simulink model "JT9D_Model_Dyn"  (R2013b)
settings: Solver=ode4  StartTime=0.0  StopTime=30  FixedStep=0.04  RelTol=1e-3
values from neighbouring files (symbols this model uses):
  MWS = setup_Inputs(MWS)    [JT9D_setup_everything_Dyn.m]    (also in JT9D_setup_everything_SS.m; Tsetup_Ambient.m = MWS; GasTurbine_Dyn_setup_everything.m = setup_Duct(MWS))
libraries: Lib_Turbo_Duct_TMATS x5, Lib_Turbo_Compressor_TMATS x3, Lib_Solve_OuterLoopIntegrator_TMATS x2, Lib_Turbo_Shaft_TMATS x2, Lib_Turbo_TurbineNPSS_TMATS x2, Lib_Turbo_Nozzle_TMATS x2, Lib_Cntrl_SimplePIcontroller_TMATS x1, Lib_Solve_IterNRSolverJC_TMATS x1, Lib_Turbo_Burner_TMATS x1, Lib_Turbo_Inlet_TMATS x1, Lib_Turbo_Splitter_TMATS x1

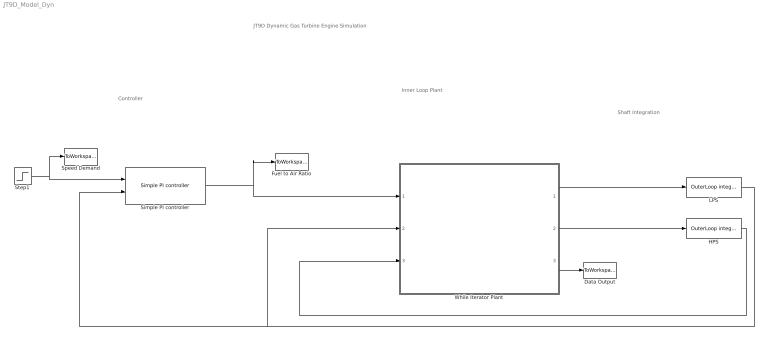
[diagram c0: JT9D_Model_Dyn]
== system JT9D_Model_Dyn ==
  note: JT9D Dynamic Gas Turbine Engine Simulation
  note: Controller
  note: Inner Loop Plant
  note: Shaft Integration
  Data Output : ToWorkspace  VariableName=Plant_Data  SampleTime=-1  SaveFormat=Timeseries
  Fuel to Air Ratio : ToWorkspace  VariableName=FAR  SampleTime=-1  SaveFormat=Timeseries
  HPS : Lib_Solve_OuterLoopIntegrator_TMATS/OuterLoop integrator  OL_IC_M=MWS.Input.HP_Shaft
  LPS : Lib_Solve_OuterLoopIntegrator_TMATS/OuterLoop integrator  OL_IC_M=MWS.Input.LP_Shaft
  Simple PI controller : Lib_Cntrl_SimplePIcontroller_TMATS/Simple PI controller  Kp_M=0.000008  Ki_M=0.00001  PI_IC_M=MWS.Input.FARin
  Speed Demand : ToWorkspace  VariableName=Nf_dmd  SampleTime=-1  SaveFormat=Timeseries
  Step1 : Step  Time=15  Before=MWS.Input.LP_Shaft  After=MWS.Input.LP_Shaft -200  SampleTime=0
  While Iterator Plant : Subsystem  TreatAsAtomicUnit=on
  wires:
  While Iterator Plant/1(LPS_Ndot) -> LPS/1
  While Iterator Plant/2(HPS_Ndot) -> HPS/1
  LPS/1 -> Simple PI controller/2, While Iterator Plant/2(LPS_NmechIn)
  HPS/1 -> While Iterator Plant/3(HPS_NmechIn)
  Simple PI controller/1 -> Fuel to Air Ratio/1, While Iterator Plant/1(FAR_Wf)
  Step1/1 -> Speed Demand/1, Simple PI controller/1
  While Iterator Plant/3(Plant_Data) -> Data Output/1

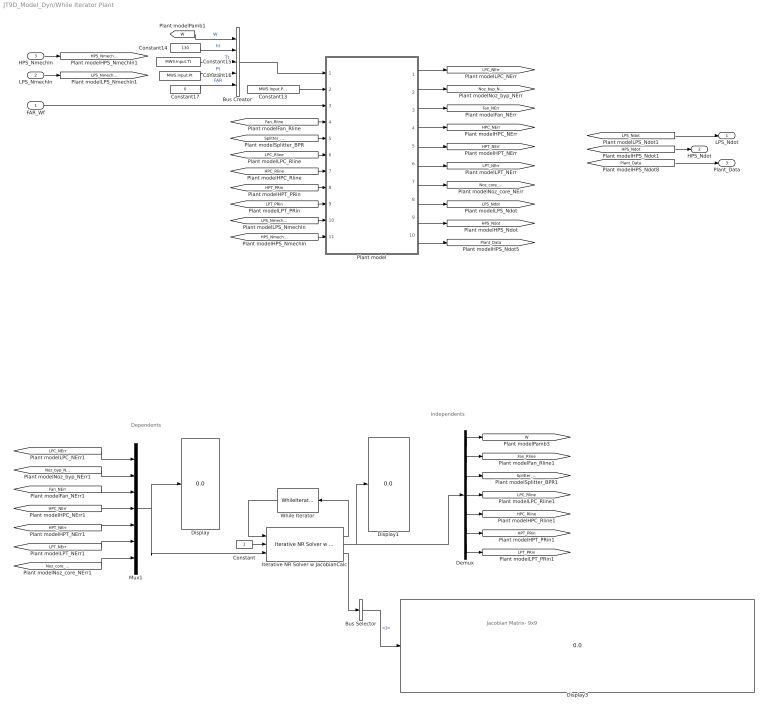
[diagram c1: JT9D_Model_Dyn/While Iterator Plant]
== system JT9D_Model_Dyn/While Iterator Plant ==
  note: Jacobian Matrix- 9x9
  note: Dependents
  note: Independents
  FAR_Wf : Inport
  LPS_NmechIn : Inport  Port=2
  HPS_NmechIn : Inport  Port=3
  Bus Creator : BusCreator  Inputs=5
  Bus Selector : BusSelector  OutputSignals=J
  Constant : Constant
  Constant13 : Constant  Value=MWS.Input.Pamb
  Constant14 : Constant  Value=130
  Constant15 : Constant  Value=MWS.Input.Tt
  Constant16 : Constant  Value=MWS.Input.Pt
  Constant17 : Constant  Value=0
  Demux : Demux  Outputs=7
  Display : Display
  Display1 : Display
  Display3 : Display
  Iterative NR Solver w JacobianCalc : Lib_Solve_IterNRSolverJC_TMATS/Iterative NR Solver w JacobianCalc  SJac_Per_M=[0.05 0.05 0.05 0.05 0.05 0.05 0.05]  SNR_IC_M=MWS.Input.NRICDyn  SNR_DX_M=5  SJacobianAttempts_M=20  Cond_Limits_M=0.0001
  Mux1 : Mux  Inputs=7
  Plant model : Subsystem
  While Iterator : WhileIterator  WhileBlockType=do-while  ShowIterationPort=on
  LPS_Ndot : Outport
  HPS_Ndot : Outport  Port=2
  Plant_Data : Outport  Port=3
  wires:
  [W] -> Bus Creator/1  "W"
  Bus Creator/1 -> Plant model/1(Input GPC)
  Constant17/1 -> Bus Creator/5  "FAR"
  Constant15/1 -> Bus Creator/3  "Tt"
  Constant16/1 -> Bus Creator/4  "Pt"
  Constant14/1 -> Bus Creator/2  "ht"
  Constant13/1 -> Plant model/2(Pamb)
  FAR_Wf/1 -> Plant model/3(FAR_dmd)
  [Fan_Rline] -> Plant model/4(Fan_Rline)
  [Splitter_BPR] -> Plant model/5(Splitter_BPR)
  [LPC_Rline] -> Plant model/6(LPC_Rline)
  [HPC_Rline] -> Plant model/7(HPC_Rline)
  [HPT_PRin] -> Plant model/8(HPT_PRin)
  [LPT_PRin] -> Plant model/9(LPT_PRin)
  [LPS_NmechIn] -> Plant model/10(LPS_NmechIn)
  [HPS_NmechIn] -> Plant model/11(HPS_NmechIn)
  Plant model/1(LPC_NErr) -> [LPC_NErr]
  Plant model/2(Noz_byp_NErr) -> [Noz_byp_NErr]
  Plant model/3(Fan_NErr) -> [Fan_NErr]
  Plant model/4(HPC_NErr) -> [HPC_NErr]
  Plant model/5(HPT_NErr) -> [HPT_NErr]
  Plant model/6(LPT_NErr) -> [LPT_NErr]
  Plant model/7(Noz_core_NErr) -> [Noz_core_NErr]
  Plant model/8(LPS_Ndot) -> [LPS_Ndot]
  Plant model/9(HPS_Ndot) -> [HPS_Ndot]
  Demux/1 -> [W]
  Demux/7 -> [LPT_PRin]
  Demux/5 -> [HPC_Rline]
  Demux/6 -> [HPT_PRin]
  Demux/4 -> [LPC_Rline]
  Demux/2 -> [Fan_Rline]
  Demux/3 -> [Splitter_BPR]
  [Fan_NErr] -> Mux1/3
  [HPC_NErr] -> Mux1/4
  [Noz_byp_NErr] -> Mux1/2
  [HPT_NErr] -> Mux1/5
  [LPC_NErr] -> Mux1/1
  [LPT_NErr] -> Mux1/6
  [Noz_core_NErr] -> Mux1/7
  Iterative NR Solver w JacobianCalc/3 -> Bus Selector/1
  Mux1/1 -> Iterative NR Solver w JacobianCalc/3, Display/1
  Bus Selector/1 -> Display3/1  "<J>"
  Iterative NR Solver w JacobianCalc/2 -> Demux/1, Display1/1
  Iterative NR Solver w JacobianCalc/1 -> While Iterator/1
  HPS_NmechIn/1 -> [HPS_NmechIn]
  LPS_NmechIn/1 -> [LPS_NmechIn]
  [LPS_Ndot] -> LPS_Ndot/1
  [HPS_Ndot] -> HPS_Ndot/1
  Plant model/10(Plant_Data) -> [Plant_Data]
  [Plant_Data] -> Plant_Data/1
  Constant/1 -> Iterative NR Solver w JacobianCalc/2
  While Iterator/1 -> Iterative NR Solver w JacobianCalc/1

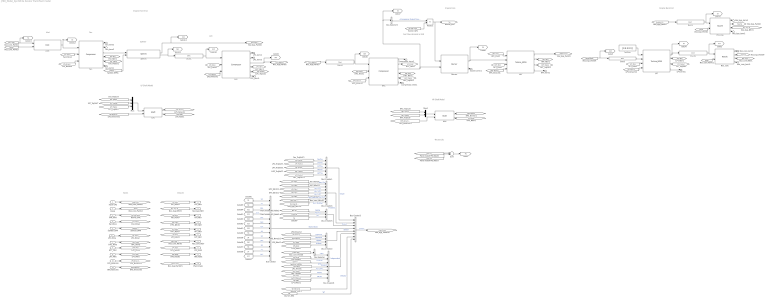
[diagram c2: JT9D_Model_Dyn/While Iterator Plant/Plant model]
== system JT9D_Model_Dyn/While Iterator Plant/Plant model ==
  note: LP Shaft Model
  note: Inputs
  note: Outputs
  note: Engine Core
  note: HP Shaft Model
  note: Engine Back End
  note: Engine Front End
  note: Fuel Flow demand as FAR
  note: Inlet
  note: Fan
  note: Splitter
  note: LPC
  note: Thrust Calc
  Input GPC : Inport
  Pamb : Inport  Port=2
  FAR_dmd : Inport  Port=3
  Fan_Rline : Inport  Port=4
  Splitter_BPR : Inport  Port=5
  LPC_Rline : Inport  Port=6
  HPC_Rline : Inport  Port=7
  HPT_PRin : Inport  Port=8
  LPT_PRin : Inport  Port=9
  LPS_NmechIn : Inport  Port=10
  HPS_NmechIn : Inport  Port=11
  Burner : Lib_Turbo_Burner_TMATS/Burner  LHV_M=18400  dPnormBurner_M=MWS.Burn.dP  Eff_M=0.994
  Burner_term1 : Terminator
  Bus Creator : BusCreator  Inputs=13
  Bus Creator1 : BusCreator  Inputs=5
  Bus Creator2 : BusCreator
  Bus Creator3 : BusCreator  Inputs=8
  Bus Creator4 : BusCreator  Inputs=7
  Bus Creator5 : BusCreator  Inputs=3
  Bus Creator6 : BusCreator  Inputs=7
  Bus Selector : BusSelector  OutputSignals=W
  Bus Selector5 : BusSelector  OutputSignals=Compressor Output Flow; WOut[pps]
  Compressor_term1 : Terminator
  Compressor_term2 : Terminator
  Duct1 : Lib_Turbo_Duct_TMATS/Duct  dP_M=MWS.Duct.dP1
  Duct2 : Lib_Turbo_Duct_TMATS/Duct  dP_M=MWS.Duct.dP2
  Duct3 : Lib_Turbo_Duct_TMATS/Duct  dP_M=MWS.Duct.dP3
  Duct4 : Lib_Turbo_Duct_TMATS/Duct  dP_M=MWS.Duct.dP4
  Duct5 : Lib_Turbo_Duct_TMATS/Duct  dP_M=MWS.Duct.dP5
  Fan : Lib_Turbo_Compressor_TMATS/Compressor  X_C_RlineVec_M=MWS.FAN.RlineVec  Y_C_NcVec_M=MWS.FAN.NcVec  T_C_Map_WcArray_M=MWS.FAN.WcArray  T_C_Map_PRArray_M=MWS.FAN.PRArray  T_C_Map_EffArray_M=MWS.FAN.EffArray  s_C_Nc_M=MWS.FAN.s_Nc  s_C_Wc_M=MWS.FAN.s_Wc  s_C_PR_M=MWS.FAN.s_PR  s_C_Eff_M=MWS.FAN.s_eff  CBLDEN_M=off  C_CBD_M=0  C_CBFht_M=0.5  C_CBFPt_M=0.5  FBLDEN_M=off  C_FBD_M=0  C_BFht_M=0.5  C_BFPt_M=0.5  X_C_WcSurgeVec_M=[0 5000]  T_C_PRSurgeVec_M=[30 30]  iDesign_M=MWS.iDes  NcDes_M=1  EffDes_M=0.8675  PRDes_M=1.645  RlineDes_M=2.3706  FVar_M='iDesScalars.mat'  SVar_M=gcb  NcNm_M='_C_Nc'  WcNm_M='_C_Wc'  PRNm_M='_C_PR'  EffNm_M='_C_Eff'
  Fan_term1 : Terminator
  Fan_term2 : Terminator
  Fan_term3 : Terminator
  HPC : Lib_Turbo_Compressor_TMATS/Compressor  X_C_RlineVec_M=MWS.HPC.RlineVec  Y_C_NcVec_M=MWS.HPC.NcVec  T_C_Map_WcArray_M=MWS.HPC.WcArray  T_C_Map_PRArray_M=MWS.HPC.PRArray  T_C_Map_EffArray_M=MWS.HPC.EffArray  s_C_Nc_M=MWS.HPC.s_Nc  s_C_Wc_M=MWS.HPC.s_Wc  s_C_PR_M=MWS.HPC.s_PR  s_C_Eff_M=MWS.HPC.s_eff  CBLDEN_M=off  C_CBD_M=0  C_CBFht_M=0.5  C_CBFPt_M=0.5  FBLDEN_M=on  C_FBD_M=MWS.HPC.Fbld  C_BFht_M=MWS.HPC.Fblde  C_BFPt_M=MWS.HPC.Fbldp  X_C_WcSurgeVec_M=[0 200]  T_C_PRSurgeVec_M=[30 30]  iDesign_M=MWS.iDes  NcDes_M=0.995  EffDes_M=.8651  PRDes_M=5.609  RlineDes_M=2.0424  FVar_M='iDesScalars.mat'  SVar_M=gcb  NcNm_M='_C_Nc'  WcNm_M='_C_Wc'  PRNm_M='_C_PR'  EffNm_M='_C_Eff'
  HPS : Lib_Turbo_Shaft_TMATS/Shaft  Shaft_Inertia_M=MWS.Shaft.Iner_hp
  HPT : Lib_Turbo_TurbineNPSS_TMATS/Turbine_NPSS  X_T_PRVec_M=MWS.HPT.PRVec  Y_T_NcVec_M=MWS.HPT.NcVec  T_T_Map_WcArray_M=MWS.HPT.WcArray  T_T_Map_EffArray_M=MWS.HPT.EffArray  s_T_Nc_M=MWS.HPT.s_Nc  s_T_Wc_M=MWS.HPT.s_Wc  s_T_PR_M=MWS.HPT.s_PR  s_T_Eff_M=MWS.HPT.s_eff  CFlwEn_M=on  T_CoolFlwPos_M=MWS.HPT.Cool  iDesign_M=MWS.iDes  NcDes_M=99.031  EffDes_M=.9133  PRDes_M=4.930  NDes_M=7390  FVar_M='iDesScalars.mat'  SVar_M=gcb  NcNm_M='_C_Nc'  WcNm_M='_C_Wc'  PRNm_M='_C_PR'  EffNm_M='_C_Eff'
  HPT_term1 : Terminator
  Inlet : Lib_Turbo_Inlet_TMATS/Inlet  eRambase_M=MWS.Inlet.eRamBase  X_eRamVec_M=MWS.Inlet.eRamVec  T_eRamtbl_M=MWS.Inlet.eRamtbl
  LPC : Lib_Turbo_Compressor_TMATS/Compressor  X_C_RlineVec_M=MWS.LPC.RlineVec  Y_C_NcVec_M=MWS.LPC.NcVec  T_C_Map_WcArray_M=MWS.LPC.WcArray  T_C_Map_PRArray_M=MWS.LPC.PRArray  T_C_Map_EffArray_M=MWS.LPC.EffArray  s_C_Nc_M=MWS.LPC.s_Nc  s_C_Wc_M=MWS.LPC.s_Wc  s_C_PR_M=MWS.LPC.s_PR  s_C_Eff_M=MWS.LPC.s_eff  CBLDEN_M=off  C_CBD_M=0  C_CBFht_M=0.5  C_CBFPt_M=0.5  FBLDEN_M=off  C_FBD_M=0  C_BFht_M=0.5  C_BFPt_M=0.5  X_C_WcSurgeVec_M=[0 200]  T_C_PRSurgeVec_M=[30 30]  iDesign_M=MWS.iDes  NcDes_M=0.993  EffDes_M=.8683  PRDes_M=2.488  RlineDes_M=1.7664  FVar_M='iDesScalars.mat'  SVar_M=gcb  NcNm_M='_C_Nc'  WcNm_M='_C_Wc'  PRNm_M='_C_PR'  EffNm_M='_C_Eff'
  LPC_term1 : Terminator
  LPC_term2 : Terminator
  LPC_term3 : Terminator
  LPS : Lib_Turbo_Shaft_TMATS/Shaft  Shaft_Inertia_M=MWS.Shaft.Iner_lp
  LPT : Lib_Turbo_TurbineNPSS_TMATS/Turbine_NPSS  X_T_PRVec_M=MWS.LPT.PRVec  Y_T_NcVec_M=MWS.LPT.NcVec  T_T_Map_WcArray_M=MWS.LPT.WcArray  T_T_Map_EffArray_M=MWS.LPT.EffArray  s_T_Nc_M=MWS.LPT.s_Nc  s_T_Wc_M=MWS.LPT.s_Wc  s_T_PR_M=MWS.LPT.s_PR  s_T_Eff_M=MWS.LPT.s_eff  CFlwEn_M=off  T_CoolFlwPos_M=0  iDesign_M=MWS.iDes  NcDes_M=105.038  EffDes_M=.9323  PRDes_M=6.420  NDes_M=3667.6  FVar_M='iDesScalars.mat'  SVar_M=gcb  NcNm_M='_C_Nc'  WcNm_M='_C_Wc'  PRNm_M='_C_PR'  EffNm_M='_C_Eff'
  LPT_term1 : Terminator
  Mux : Mux  Inputs=3
  Mux1 : Mux  Inputs=2
  NoFlow : Constant  Value=[0 0 0 0 0]
  Noz_byp : Lib_Turbo_Nozzle_TMATS/Nozzle  SWType_M=1  N_TArea_M=MWS.NozB.Ath  N_EArea_M=110.7  N_FL_M=0.00  X_N_TtVec2_M=[300 2000]  T_N_TGArray_M=[1 1]  X_N_PEQPaVec_M=[0 10000]  T_N_CdThArray_M=[1 1]  T_N_CvArray_M=MWS.NozB.CvArray  T_N_CfgArray_M=[1 1]  X_N_FARVec_M=[0; 0.0050; 0.0100; 0.0150; 0.0200; 0.0250; 0.0300]  T_N_RtArray_M="[0.0686;    0.0686;    0.0686;    0.0686;    0.0686;    0.0686;    0.0686]"  Y_N_TtVec_M=[300 2000]  T_N_MAP_gammaArray_M=[ 1.4 1.4 1.4 1.4 1.4 1.4 1.4; 1.4 1.4 1.4 1.4 1.4 1.4 1.4]  iDesign_M=MWS.iDes  WDes_M=562.61  FVar_M='iDesScalars.mat'  SVar_M=gcb  AthNm_M='_Ath'  AxNm_M='_Ax'
  Noz_byp_term1 : Terminator
  Noz_byp_term3 : Terminator
  Noz_core : Lib_Turbo_Nozzle_TMATS/Nozzle  SWType_M=1  N_TArea_M=MWS.Noz.Ath  N_EArea_M=110.7  N_FL_M=0.00  X_N_TtVec2_M=[300 2000]  T_N_TGArray_M=[1 1]  X_N_PEQPaVec_M=[0 10000]  T_N_CdThArray_M=[1 1]  T_N_CvArray_M=MWS.Noz.CvArray  T_N_CfgArray_M=[1 1]  X_N_FARVec_M=[0; 0.0050; 0.0100; 0.0150; 0.0200; 0.0250; 0.0300]  T_N_RtArray_M="[0.0686;    0.0686;    0.0686;    0.0686;    0.0686;    0.0686;    0.0686]"  Y_N_TtVec_M=[300 2000]  T_N_MAP_gammaArray_M=[ 1.4 1.4 1.4 1.4 1.4 1.4 1.4; 1.4 1.4 1.4 1.4 1.4 1.4 1.4]  iDesign_M=MWS.iDes  WDes_M=113.51  FVar_M='iDesScalars.mat'  SVar_M=gcb  AthNm_M='_Ath'  AxNm_M='_Ax'
  Noz_core_term1 : Terminator
  Noz_core_term2 : Terminator
  Product : Product
  Splitter : Lib_Turbo_Splitter_TMATS/Splitter
  Sum : Sum  Inputs=|++
  LPC_NErr : Outport
  Noz_byp_NErr : Outport  Port=2
  Fan_NErr : Outport  Port=3
  HPC_NErr : Outport  Port=4
  HPT_NErr : Outport  Port=5
  LPT_NErr : Outport  Port=6
  Noz_core_NErr : Outport  Port=7
  LPS_Ndot : Outport  Port=8
  HPS_Ndot : Outport  Port=9
  Plant_Data : Outport  Port=10
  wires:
  Fan_Rline/1 -> [Fan_Rline]
  HPS_NmechIn/1 -> [HPS_NmechIn]
  HPC_Rline/1 -> [HPC_Rline]
  LPT_PRin/1 -> [LPT_PRin]
  FAR_dmd/1 -> [Wf_FAR_dmd]
  Splitter_BPR/1 -> [Splitter_BPR]
  LPC_Rline/1 -> [LPC_Rline]
  HPT_PRin/1 -> [HPT_PRin]
  LPS_NmechIn/1 -> [LPS_NmechIn]
  Duct1/1 -> [S22], LPC/1
  Duct4/1 -> [S17], Noz_core/1
  HPC/6 -> Compressor_term1/1
  Noz_core/4 -> Noz_core_term1/1
  [Pamb] -> Noz_core/2
  Noz_core/3 -> [Noz_core_NErr]
  Duct3/1 -> LPT/2
  Noz_core/2 -> [Core_Fg]
  Mux/1 -> LPS/1
  Mux1/1 -> HPS/1
  [LPT_TrqOut] -> Mux/3
  [Fan_TrqOut] -> Mux/1
  [HPT_TrqOut] -> Mux1/2
  [HPC_TrqOut] -> Mux1/1
  [LPC_TrqOut] -> Mux/2
  HPS/2 -> [HPS_Ndot]
  HPS/1 -> [HPS_Nmech]
  [LPS_Nmech] -> Fan/3
  [LPS_Nmech] -> LPT/4
  [HPS_NmechIn] -> HPS/2
  [HPS_Nmech] -> HPC/3
  [LPS_Nmech] -> LPC/3
  Duct5/1 -> [S7], Noz_byp/1
  LPT/2 -> [LPT_NErr]
  [LPT_PRin] -> LPT/3
  LPT/4 -> LPT_term1/1
  [HPS_Nmech] -> HPT/4
  LPS/2 -> [LPS_Ndot]
  LPS/1 -> [LPS_Nmech]
  [LPS_NmechIn] -> LPS/2
  HPT/4 -> HPT_term1/1
  Splitter/2 -> [S21], Duct1/1
  Fan/3 -> Splitter/1
  Splitter/1 -> [S13], [BypassFlowOut]
  Burner/1 -> HPT/2, [S4]
  LPT/1 -> [S5], Duct4/1
  HPC/3 -> [S3], Bus Selector5/1, Burner/2
  LPC/3 -> [S23], [LPCFlowOut]
  HPT/2 -> [HPT_NErr]
  [HPT_PRin] -> HPT/3
  NoFlow/1 -> LPT/1
  Inlet/1 -> [S2], Fan/1
  LPT/3 -> [LPT_TrqOut]
  HPC/1 -> Compressor_term2/1
  Noz_byp/3 -> [Noz_byp_NErr]
  [Fan_Rline] -> Fan/2
  Noz_byp/1 -> Noz_byp_term3/1
  HPT/3 -> [HPT_TrqOut]
  Noz_byp/4 -> Noz_byp_term1/1
  [Pamb] -> Noz_byp/2
  Noz_byp/2 -> [Byp_Fg]
  Burner/2 -> Burner_term1/1
  LPC/2 -> LPC_term3/1
  LPC/4 -> [LPC_NErr]
  LPC/1 -> LPC_term2/1
  LPC/5 -> [LPC_TrqOut]
  [LPC_Rline] -> LPC/2
  [Splitter_BPR] -> Splitter/2
  [HPC_Fbld] -> HPT/1
  Fan/5 -> [Fan_TrqOut]
  Fan/4 -> [Fan_NErr]
  Fan/2 -> Fan_term3/1
  Fan/6 -> Fan_term1/1
  Fan/1 -> Fan_term2/1
  HPC/5 -> [HPC_TrqOut]
  [HPC_Rline] -> HPC/2
  HPC/4 -> [HPC_NErr]
  HPC/2 -> [HPC_Fbld]
  LPC/6 -> LPC_term1/1
  [LPC_NErr] -> LPC_NErr/1
  [Noz_byp_NErr] -> Noz_byp_NErr/1
  [Fan_NErr] -> Fan_NErr/1
  [HPC_NErr] -> HPC_NErr/1
  [HPT_NErr] -> HPT_NErr/1
  [LPT_NErr] -> LPT_NErr/1
  [Noz_core_NErr] -> Noz_core_NErr/1
  [LPS_Ndot] -> LPS_Ndot/1
  [HPS_Ndot] -> HPS_Ndot/1
  [HPTFlowOut] -> [S45], Duct3/1
  [Wf_FAR_dmd] -> Product/2
  Bus Selector5/1 -> Product/1  "<Compressor Output Flow; WOut[pps]>"
  Product/1 -> [Wf], Burner/1
  Pamb/1 -> [Pamb]
  [Pamb] -> Inlet/2
  [Input_GPC] -> [S1], Inlet/1
  Input GPC/1 -> [Input_GPC]
  Noz_core/1 -> Noz_core_term2/1
  [LPCFlowOut] -> Duct2/1
  HPT/1 -> [HPTFlowOut]
  [BypassFlowOut] -> Duct5/1
  [Plant_Data] -> Plant_Data/1
  [S23] -> Bus Creator/6  "S23"
  [S22] -> Bus Creator/5  "S22"
  [S24] -> Bus Creator/7  "S24"
  [S3] -> Bus Creator/8  "S3"
  [S13] -> Bus Creator/4  "S13"
  [S4] -> Bus Creator/9  "S4"
  [S21] -> Bus Creator/3  "S21"
  [S45] -> Bus Creator/10  "S45"
  [S2] -> Bus Creator/2  "S2"
  [S1] -> Bus Creator/1  "S1"
  [S5] -> Bus Creator/11  "S5"
  [S7] -> Bus Creator/12  "S7"
  [S17] -> Bus Creator/13  "S17"
  Bus Creator/1 -> Bus Creator3/4  "StationData"
  Bus Creator2/1 -> Bus Creator3/5  "Speed"
  Bus Creator1/1 -> Bus Creator3/1  "Torque"
  Bus Creator3/1 -> [Plant_Data]  "Output"
  [Fan_NErr] -> Bus Creator4/1  "Nerr_Fan"
  [Noz_byp_NErr] -> Bus Creator4/7  "Nerr_NozByp"
  [LPC_NErr] -> Bus Creator4/2  "Nerr_LPC"
  [HPC_NErr] -> Bus Creator4/3  "Nerr_HPC"
  [HPT_NErr] -> Bus Creator4/4  "Nerr_HPT"
  [LPT_NErr] -> Bus Creator4/5  "Nerr_LPT"
  [Noz_core_NErr] -> Bus Creator4/6  "Nerr_NozCore"
  [Fan_TrqOut] -> Bus Creator1/1  "FanTrq"
  [LPC_TrqOut] -> Bus Creator1/2  "LPCTrq"
  [HPC_TrqOut] -> Bus Creator1/4  "HPCTrq"
  [HPT_TrqOut] -> Bus Creator1/5  "HPTTrq"
  [LPT_TrqOut] -> Bus Creator1/3  "LPTTrq"
  [Byp_Fg] -> Bus Creator5/1  "BypFg"
  [Core_Fg] -> Bus Creator5/2  "MainFg"
  [Fg] -> Bus Creator5/3  "Fg"
  [LPS_Nmech] -> Bus Creator2/1  "LPSpeed"
  [HPS_Nmech] -> Bus Creator2/2  "HPSpeed"
  [LPS_Ndot] -> Bus Creator2/3  "LPNdot"
  [HPS_Ndot] -> Bus Creator2/4  "HPNdot"
  [HPT_PRin] -> Bus Creator6/6  "PRHPT"
  [HPC_Rline] -> Bus Creator6/5  "RlineHPC"
  [Fan_Rline] -> Bus Creator6/2  "RlineFan"
  [Splitter_BPR] -> Bus Creator6/3  "BPR"
  [LPC_Rline] -> Bus Creator6/4  "RlineLPC"
  [LPT_PRin] -> Bus Creator6/7  "PRLPT"
  Bus Selector/1 -> Bus Creator6/1  "<W>"
  Bus Creator4/1 -> Bus Creator3/2  "FlowError"
  Bus Creator5/1 -> Bus Creator3/3  "Thrust"
  Bus Creator6/1 -> Bus Creator3/6  "Independents"
  [Wf_FAR_dmd] -> Bus Creator3/7  "FARdmd"
  [Byp_Fg] -> Sum/1
  [Core_Fg] -> Sum/2
  Sum/1 -> [Fg]
  Duct2/1 -> [S24], HPC/1
  [Wf] -> Bus Creator3/8  "Wf"
  [Input_GPC] -> Bus Selector/1
